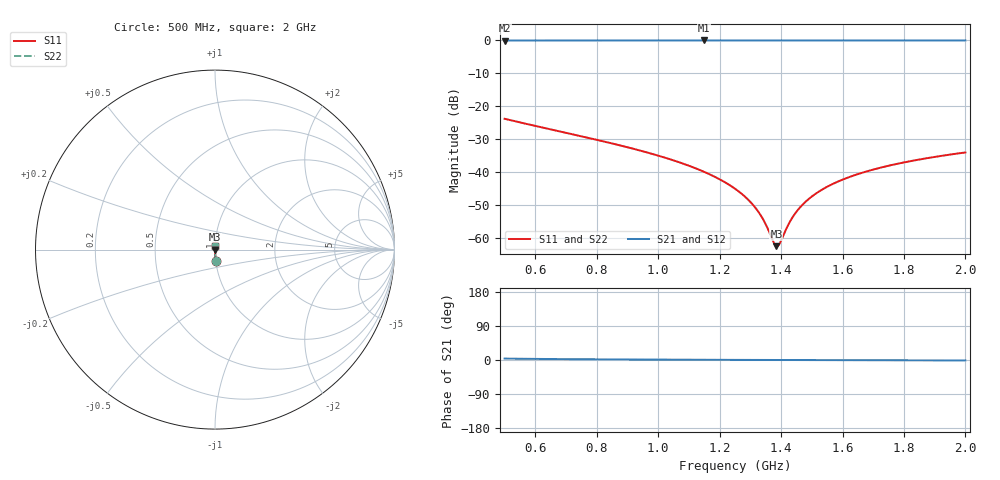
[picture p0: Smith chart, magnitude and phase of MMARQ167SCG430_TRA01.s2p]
! MMARQ167SCG430_TRA01  S-PARAMETER MODEL  ( General Type )
! Model Generated by TAIYO YUDEN Corporation (http://www.ty-top.com)
! Version 1.0
! TAIYO YUDEN Control No. 160201
! Copyright(c) 2016 TAIYO YUDEN CO.,LTD. All Rights Reserved.
! Product Description (link to TY-COMPAS)
! https://ds.yuden.co.jp/TYCOMPAS/or/detail?pn=MMARQ167SCG430JTRA01&u=M
! Products Name : Multilayer Ceramic Capacitors
! Characteristics :
!  Capacitance : 43 pF , Rated Voltage : 250V , TCC : CG / C0G
!  Case Size : 1.6 x 0.8 / 0.063 x 0.031 [mm/inch] , Thickness : 0.7 / 0.028 [mm/inch]
!  (Conditions: Temperature = 25 degC , DC Bias Current/Voltage = 0A / 0V)
! External Node Assignments :
!  1  o---| |---o  2
! GND o---------o GND
! Frequency Range : 500MHz  -  2000MHz  [ 401 STEP ]
# MHz S RI R 50
! Freq[MHz].  S11 Real  S11 Imag  S21 Real  S21 Imag  S12 Real  S12 Imag  S22 Real  S22 Imag
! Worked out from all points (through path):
!   401 points, 500 MHz to 2 GHz, reference 50 ohm
!   highest |S21| = -0.01 dB at 1.149 GHz (marker M1); lowest = 0.0 dB at 500 MHz (marker M2)
!   lowest |S11| = -62.6 dB at 1.385 GHz (marker M3), VSWR 1.00, Z = 50.1 - j0.00693 ohm
!   |S11| at or under -10 dB: start of sweep to end of sweep
!   |S22| runs from -62.6 to -23.8 dB; largest |S21 - S12| = 0
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500  0.00443 -0.0642  0.9956 0.0642  0.9956 0.0642  0.00443 -0.0642
751.25  0.00163 -0.0347  0.9984 0.0347  0.9984 0.0347  0.00163 -0.0347
1002.5  0.000872 -0.0176  0.9991 0.0176  0.9991 0.0176  0.000872 -0.0176
1148.75  0.000738 -0.0101  0.9993 0.0101  0.9993 0.0101  0.000738 -0.0101
1205  0.000719 -0.00748  0.9993 0.00748  0.9993 0.00748  0.000719 -0.00748
1250  0.000714 -0.00552  0.9993 0.00552  0.9993 0.00552  0.000714 -0.00552
1291.25  0.000716 -0.00379  0.9993 0.00379  0.9993 0.00379  0.000716 -0.00379
1321.25  0.000721 -0.00257  0.9993 0.00257  0.9993 0.00257  0.000721 -0.00257
1347.5  0.000728 -0.00152  0.9993 0.00152  0.9993 0.00152  0.000728 -0.00152
1377.5  0.000738 -0.000357  0.9993 0.000357  0.9993 0.000357  0.000738 -0.000357
1385  0.000741 -6.92e-05  0.9993 6.92e-05  0.9993 6.92e-05  0.000741 -6.92e-05
1396.25  0.000745 0.000359  0.9993 -0.000359  0.9993 -0.000359  0.000745 0.000359
1422.5  0.000757 0.00135  0.9992 -0.00135  0.9992 -0.00135  0.000757 0.00135
1445  0.000769 0.00218  0.9992 -0.00218  0.9992 -0.00218  0.000769 0.00218
1471.25  0.000784 0.00313  0.9992 -0.00313  0.9992 -0.00313  0.000784 0.00313
1501.25  0.000803 0.0042  0.9992 -0.0042  0.9992 -0.0042  0.000803 0.0042
1546.25  0.000835 0.00577  0.9992 -0.00577  0.9992 -0.00577  0.000835 0.00577
1602.5  0.00088 0.00767  0.9991 -0.00767  0.9991 -0.00767  0.00088 0.00767
1670  0.000941 0.00988  0.9991 -0.00988  0.9991 -0.00988  0.000941 0.00988
1752.5  0.00102 0.0125  0.999 -0.0125  0.999 -0.0125  0.00102 0.0125
1868.75  0.00116 0.016  0.9988 -0.016  0.9988 -0.016  0.00116 0.016
2000  0.00133 0.0197  0.9987 -0.0197  0.9987 -0.0197  0.00133 0.0197
